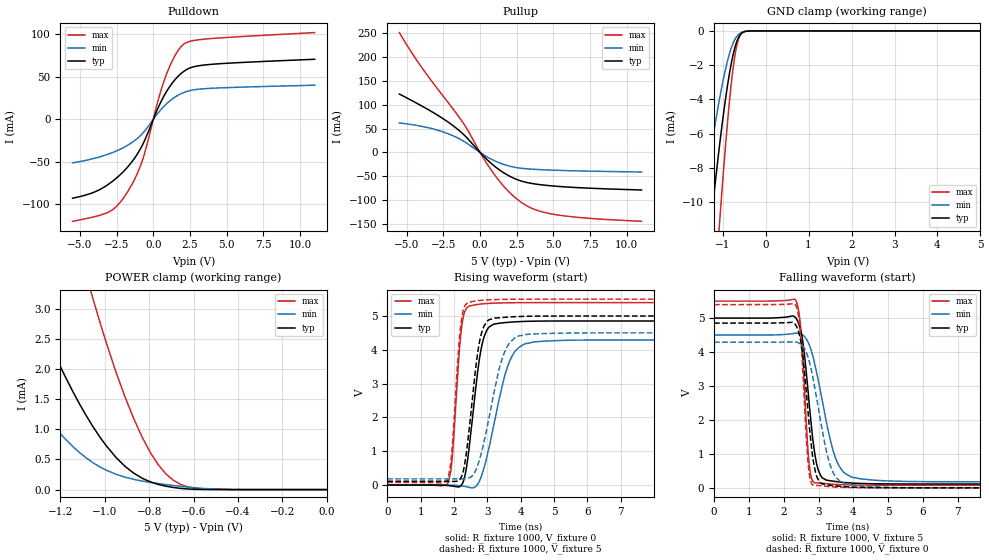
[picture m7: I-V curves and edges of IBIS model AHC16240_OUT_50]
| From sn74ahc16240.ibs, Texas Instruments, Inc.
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[Model]   AHC16240_OUT_50
Model_type  3-state
Enable   Active-Low
Vref =   0
Rref =   1000
Cref =   50p
Vmeas =   2.5
| variable   typ   min   max
C_comp   2.74pF   2.26pF   3.03pF
| C_pullup   3.76pF   2.48pF   4.89pF
| C_pulldown   3.31pF   2.65pF   4.20pF
| C_tri-state   2.74pF   2.26pF   3.03pF
[Temperature Range]   40   100   -40
| Ambient temperature   25   85   -40
[Voltage range]   5   4.5   5.5
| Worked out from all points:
|   slope of the pulldown table from 0 to 0.75 V, typ, clamps not added: 26.6 ohm
|   slope of the pullup table from 0 to 0.75 V, typ, clamps not added: 33.1 ohm
|   GND clamp passes 1 mA (typ) near -0.72 V on its own axis
|   POWER clamp passes 1 mA (typ) near -1.05 V on its own axis
|   rising waveform, R_fixture 1000, V_fixture 0: 20-80 % time 351ps typ, 592ps min, 223ps max; typ from 0 V to 4.85 V
|   falling waveform, R_fixture 1000, V_fixture 5: 20-80 % time 296ps typ, 541ps min, 180ps max; typ from 5 V to 0.112 V
|   rising waveform, R_fixture 1000, V_fixture 5: 20-80 % time 339ps typ, 569ps min, 220ps max; typ from 0.112 V to 5 V
|   falling waveform, R_fixture 1000, V_fixture 0: 20-80 % time 276ps typ, 479ps min, 176ps max; typ from 4.85 V to 0 V
[GND Clamp]
| AHC16240_OUT_50
|   Voltage   I(typ)   I(min)   I(max)
-5.5V     -169.3mA   -111.2mA   -212.8mA
-1.545V   -18.47mA   -11.66mA   -29.3mA
-1.49V    -16.94mA   -10.66mA   -27.06mA
-1.265V   -11.08mA   -6.838mA   -18.23mA
-1.085V   -6.949mA   -4.144mA   -11.67mA
-1.06V    -6.423mA   -3.803mA   -10.81mA
-915mV    -3.656mA   -2.037mA   -6.158mA
-840mV    -2.461mA   -1.314mA   -4.078mA
-765mV    -1.48mA    -761.6uA   -2.341mA
-655mV    -517uA     -273.9uA   -686uA
-545mV    -107.3uA   -73.68uA   -106.2uA
5V        48.57nA    6.899uA    454.2nA
[POWER Clamp]
| AHC16240_OUT_50
|   Voltage   I(typ)   I(min)   I(max)
-5.5V     86.69mA    55.4mA     139.9mA
-1.62V    6.126mA    3.297mA    12.91mA
-1.585V   5.725mA    3.057mA    12.18mA
-1.34V    3.216mA    1.58mA     7.528mA
-1.18V    1.886mA    846.4uA    4.929mA
-1.055V   1.054mA    450.5uA    3.187mA
-950mV    534.9uA    254.5uA    1.953mA
-870mV    273.4uA    170.2uA    1.179mA
-795mV    128.9uA    119.3uA    614.9uA
-690mV    34.77uA    67.54uA    151.5uA
-555mV    1.883uA    18.6uA     9.964uA
-95.1fV   48.57nA    2.7nA      695.6nA
[Pulldown]
| AHC16240_OUT_50
|   Voltage   I(typ)   I(min)   I(max)
-5.5V     -92.74mA   -51.13mA   -119.9mA
-4.055V   -85.78mA   -45.98mA   -114.7mA
-2.985V   -75.45mA   -40.34mA   -108.5mA
-2.4V     -67.37mA   -36.26mA   -100.4mA
-1.755V   -56.16mA   -30.5mA    -85.32mA
-730mV    -29.9mA    -16.48mA   -47.69mA
350mV     14.43mA    8.043mA    23.82mA
895mV     32.54mA    18.23mA    52.98mA
1.495V    47.09mA    26.44mA    75.64mA
2.06V     56.3mA     31.56mA    88.33mA
3.74V     64.53mA    36.44mA    94.9mA
11V       70.8mA     40.28mA    102.2mA
[Pullup]
| AHC16240_OUT_50
|   Voltage   I(typ)   I(min)   I(max)
-5.5V     122.1mA    61.67mA    250.7mA
-4.005V   97.68mA    54.72mA    179mA
-1.84V    55.96mA    34.8mA     90.86mA
-940mV    31.99mA    19.94mA    51.56mA
120mV     -3.964mA   -2.478mA   -6.276mA
860mV     -25.56mA   -15.55mA   -41.4mA
1.72V     -44.64mA   -26.18mA   -74.46mA
2.58V     -57.41mA   -32.19mA   -99.18mA
3.635V    -65.41mA   -35.15mA   -118.2mA
4.995V    -70.2mA    -37.1mA    -129.3mA
7.275V    -74.5mA    -38.98mA   -137.3mA
11V       -78.5mA    -40.86mA   -144mA
[Ramp]
| AHC16240_OUT_50
| variable   typ   min   max
dV/dt_r   2.95/3.62E-10   2.63/6.19E-10   3.25/2.25E-10
dV/dt_f   2.97/3.09E-10   2.63/5.55E-10   3.29/1.84E-10
R_load = 1000
[Rising Waveform]
| AHC16240_OUT_50
R_fixture =   1000
C_fixture =   0
L_fixture =   0
V_fixture =   0
V_fixture_min = 0
V_fixture_max = 0
|   Time   V(typ)   V(min)   V(max)
0s        230.9pV    442pV      108.2pV
1.81ns    -13.7mV    -3.154mV   39.21mV
1.94ns    -28.09mV   -5.765mV   724.9mV
2.155ns   -54.63mV   -19.16mV   3.883V
2.27ns    74.16mV    -32.34mV   4.916V
2.82ns    4.044V     252.1mV    5.357V
3.055ns   4.675V     1.123V     5.375V
3.655ns   4.816V     3.624V     5.392V
4.45ns    4.849V     4.239V     5.397V
50ns      4.853V     4.289V     5.397V
[Falling Waveform]
| AHC16240_OUT_50
R_fixture =   1000
C_fixture =   0
L_fixture =   0
V_fixture =   5
V_fixture_min = 4.5
V_fixture_max = 5.5
|   Time   V(typ)   V(min)   V(max)
0s        5V         4.5V       5.5V
2.355ns   4.994V     4.558V     5.505V
2.5ns     4.588V     4.53V      4.592V
2.595ns   3.932V     4.457V     2.963V
2.73ns    2.492V     4.222V     718.8mV
2.895ns   991.8mV    3.625V     141.6mV
3.1ns     302.6mV    2.608V     136.8mV
3.565ns   175.7mV    696mV      96.33mV
4.565ns   119.3mV    227mV      76.77mV
50ns      112.4mV    181.3mV    74.33mV
[Rising Waveform]
| AHC16240_OUT_50
R_fixture =   1000
C_fixture =   0
L_fixture =   0
V_fixture =   5
V_fixture_min = 4.5
V_fixture_max = 5.5
|   Time   V(typ)   V(min)   V(max)
0s        112.4mV    181.3mV    74.33mV
1.81ns    107.3mV    182mV      154.7mV
1.925ns   106.3mV    182.3mV    842mV
2.15ns    131.3mV    184.6mV    4.175V
2.245ns   292.1mV    186.5mV    5.012V
2.75ns    4.144V     698.5mV    5.458V
3.005ns   4.851V     1.757V     5.478V
3.505ns   4.961V     3.896V     5.494V
4.23ns    4.994V     4.462V     5.5V
50ns      5V         4.5V       5.5V
[Falling Waveform]
| AHC16240_OUT_50
R_fixture =   1000
C_fixture =   0
L_fixture =   0
V_fixture =   0
V_fixture_min = 0
V_fixture_max = 0
|   Time   V(typ)   V(min)   V(max)
0s        4.853V     4.289V     5.397V
2.35ns    4.791V     4.298V     5.369V
2.49ns    4.316V     4.229V     4.425V
2.635ns   2.981V     4.026V     1.693V
2.71ns    2.1V       3.806V     612.9mV
2.885ns   591.8mV    2.987V     64.74mV
3.215ns   85.15mV    1.123V     43.88mV
3.44ns    62.9mV     410mV      26.3mV
4.435ns   7.816mV    39.43mV    3.231mV
50ns      45.65nV    27.92nV    9.293nV
